(* Logix 5000 AddOnInstructionDefinition export Banner_QS18E_PD_v4; software revision 33.00 *)

TYPE Banner_QS18E_PDIO_v4 :   // Process Data for a QS18E sensors. This will include event information.
STRUCT
   Output_State : SINT;   // 0 = Inactive, 1 = Active
   Health_Signal : SINT;   // 0 = Marginal or Worse, 1 = Healthy
   Marginal_Light_State : SINT;   // 1 = Sensor is Marginal Light
   Marginal_Dark_State : SINT;   // 1 = Sensor is Marginal Dark
   Normalized_Signal_Strength : INT;
   Signal : DINT;   // Raw ADC Value
   Count : DINT;   // The output event count
   Duration : DINT;   // The output event duration
   Events_per_Minute : DINT;
   Emitter_LED : SINT;   // 0 = LED Emitter On, 1 = LED Emitter Off.
   Emitter_Status : SINT;   // 0 = Emitter enabled, 1 = Emitter disabled. Only active on QS18EK6E and QS18EK6EV models.
   PDI_DT : SINT[6];
   PDO_DT : SINT[2];
END_STRUCT
END_TYPE

ADD_ON_INSTRUCTION Banner_QS18E_PD_v4   (* revision 4.0, vendor Banner Engineering *)
// Take raw process data and convert it to usable values.
// Revision note:
// Added functionality for Emitter and Reciever QS18E models.
VAR_IN_OUT
   Process_Data : Banner_QS18E_PDIO_v4; {required}
END_VAR
VAR_INPUT
   PDI_Configuration : SINT; {required}
   Byte_Swap : BOOL; {required}
END_VAR
VAR
   Temp_iByte : SINT[4]; {access None}
END_VAR

ROUTINE Logic   (* ladder *)
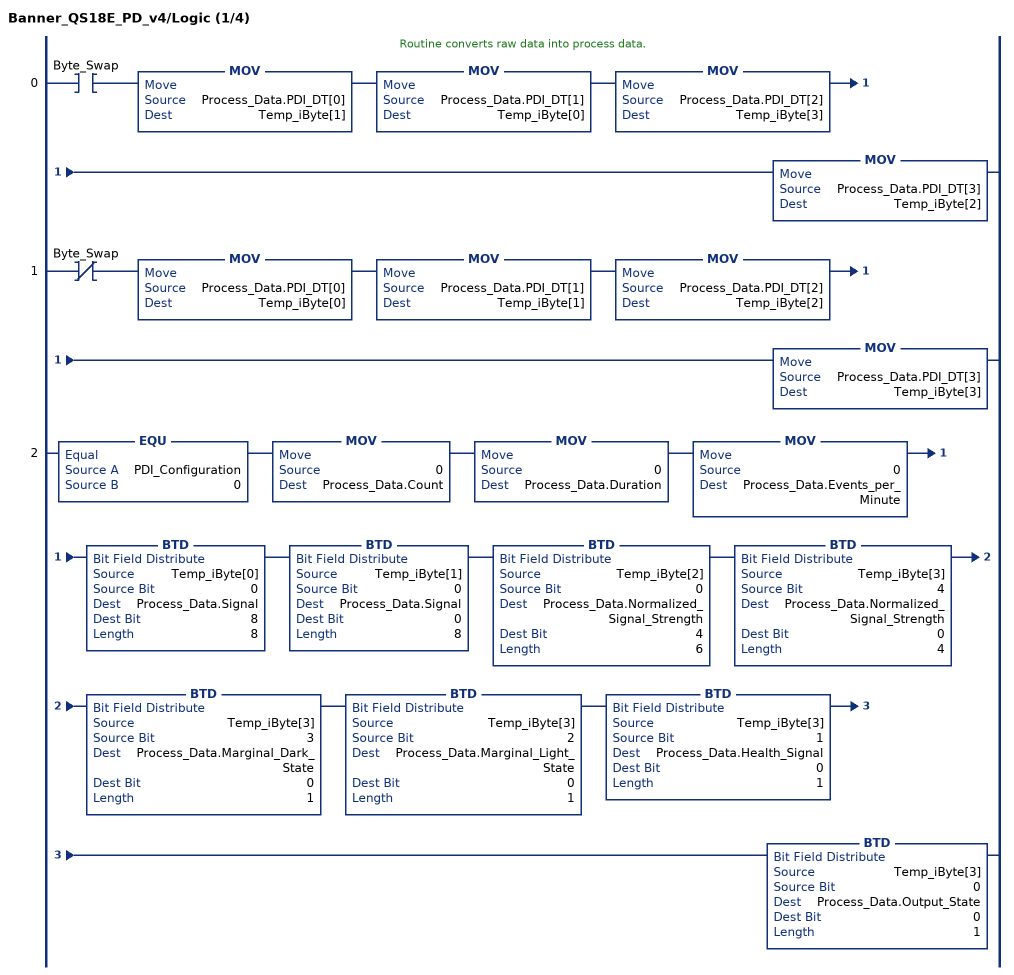
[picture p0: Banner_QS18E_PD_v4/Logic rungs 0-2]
   // Routine converts raw data into process data.
   0: XIC(Byte_Swap)MOV(Process_Data.PDI_DT[0],Temp_iByte[1])MOV(Process_Data.PDI_DT[1],Temp_iByte[0])MOV(Process_Data.PDI_DT[2],Temp_iByte[3])MOV(Process_Data.PDI_DT[3],Temp_iByte[2]);
   1: XIO(Byte_Swap)MOV(Process_Data.PDI_DT[0],Temp_iByte[0])MOV(Process_Data.PDI_DT[1],Temp_iByte[1])MOV(Process_Data.PDI_DT[2],Temp_iByte[2])MOV(Process_Data.PDI_DT[3],Temp_iByte[3]);
   2: EQU(PDI_Configuration,0)MOV(0,Process_Data.Count)MOV(0,Process_Data.Duration)MOV(0,Process_Data.Events_per_Minute)BTD(Temp_iByte[0],0,Process_Data.Signal,8,8)BTD(Temp_iByte[1],0,Process_Data.Signal,0,8)BTD(Temp_iByte[2],0,Process_Data.Normalized_Signal_Strength,4,6)BTD(Temp_iByte[3],4,Process_Data.Normalized_Signal_Strength,0,4)BTD(Temp_iByte[3],3,Process_Data.Marginal_Dark_State,0,1)BTD(Temp_iByte[3],2,Process_Data.Marginal_Light_State,0,1)BTD(Temp_iByte[3],1,Process_Data.Health_Signal,0,1)BTD(Temp_iByte[3],0,Process_Data.Output_State,0,1);
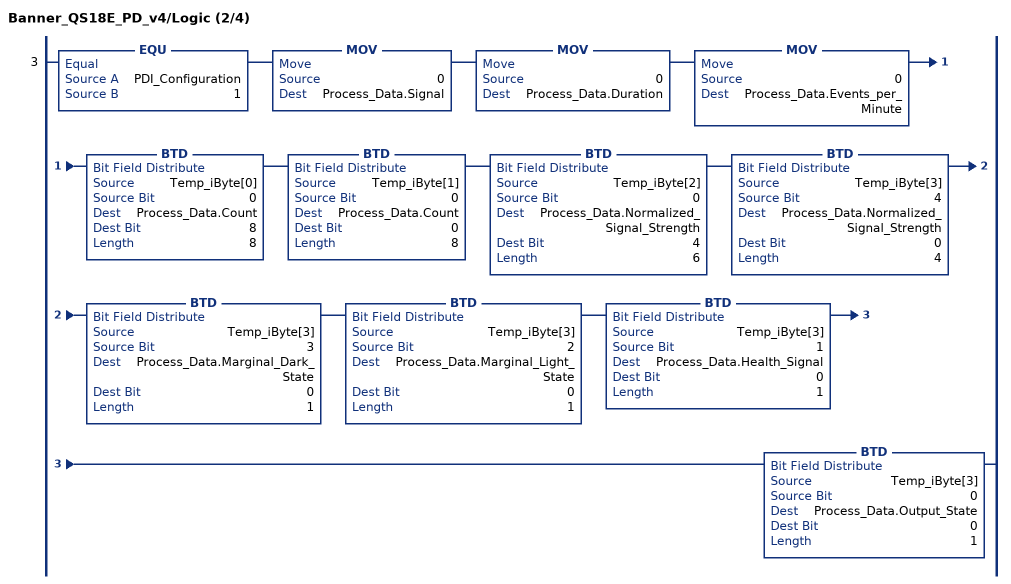
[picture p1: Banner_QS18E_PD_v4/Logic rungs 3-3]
   3: EQU(PDI_Configuration,1)MOV(0,Process_Data.Signal)MOV(0,Process_Data.Duration)MOV(0,Process_Data.Events_per_Minute)BTD(Temp_iByte[0],0,Process_Data.Count,8,8)BTD(Temp_iByte[1],0,Process_Data.Count,0,8)BTD(Temp_iByte[2],0,Process_Data.Normalized_Signal_Strength,4,6)BTD(Temp_iByte[3],4,Process_Data.Normalized_Signal_Strength,0,4)BTD(Temp_iByte[3],3,Process_Data.Marginal_Dark_State,0,1)BTD(Temp_iByte[3],2,Process_Data.Marginal_Light_State,0,1)BTD(Temp_iByte[3],1,Process_Data.Health_Signal,0,1)BTD(Temp_iByte[3],0,Process_Data.Output_State,0,1);
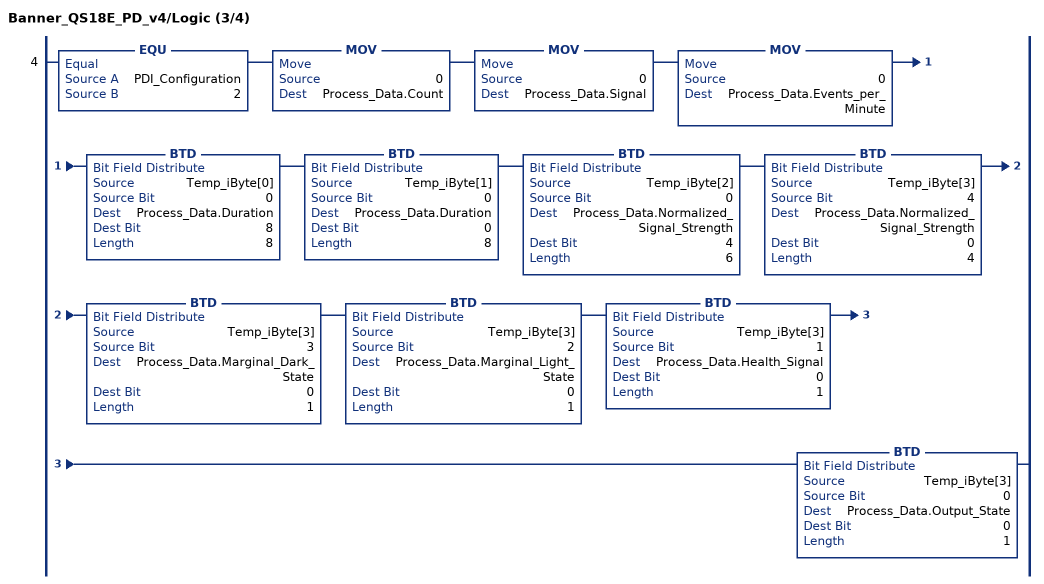
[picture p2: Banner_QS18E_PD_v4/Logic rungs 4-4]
   4: EQU(PDI_Configuration,2)MOV(0,Process_Data.Count)MOV(0,Process_Data.Signal)MOV(0,Process_Data.Events_per_Minute)BTD(Temp_iByte[0],0,Process_Data.Duration,8,8)BTD(Temp_iByte[1],0,Process_Data.Duration,0,8)BTD(Temp_iByte[2],0,Process_Data.Normalized_Signal_Strength,4,6)BTD(Temp_iByte[3],4,Process_Data.Normalized_Signal_Strength,0,4)BTD(Temp_iByte[3],3,Process_Data.Marginal_Dark_State,0,1)BTD(Temp_iByte[3],2,Process_Data.Marginal_Light_State,0,1)BTD(Temp_iByte[3],1,Process_Data.Health_Signal,0,1)BTD(Temp_iByte[3],0,Process_Data.Output_State,0,1);
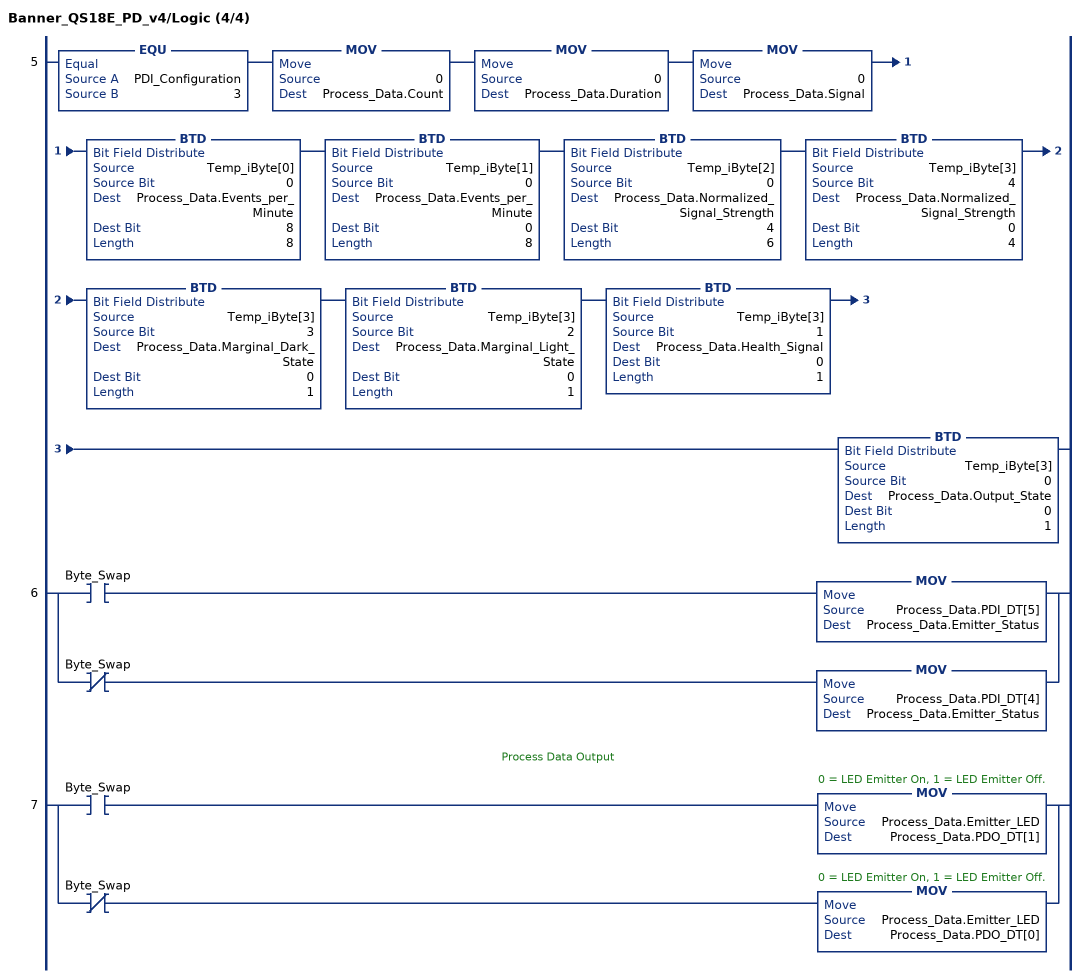
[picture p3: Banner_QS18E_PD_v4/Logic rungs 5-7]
   5: EQU(PDI_Configuration,3)MOV(0,Process_Data.Count)MOV(0,Process_Data.Duration)MOV(0,Process_Data.Signal)BTD(Temp_iByte[0],0,Process_Data.Events_per_Minute,8,8)BTD(Temp_iByte[1],0,Process_Data.Events_per_Minute,0,8)BTD(Temp_iByte[2],0,Process_Data.Normalized_Signal_Strength,4,6)BTD(Temp_iByte[3],4,Process_Data.Normalized_Signal_Strength,0,4)BTD(Temp_iByte[3],3,Process_Data.Marginal_Dark_State,0,1)BTD(Temp_iByte[3],2,Process_Data.Marginal_Light_State,0,1)BTD(Temp_iByte[3],1,Process_Data.Health_Signal,0,1)BTD(Temp_iByte[3],0,Process_Data.Output_State,0,1);
   6: [XIC(Byte_Swap) MOV(Process_Data.PDI_DT[5],Process_Data.Emitter_Status) ,XIO(Byte_Swap) MOV(Process_Data.PDI_DT[4],Process_Data.Emitter_Status) ];
   // Process Data Output
   7: [XIC(Byte_Swap) MOV(Process_Data.Emitter_LED,Process_Data.PDO_DT[1]) ,XIO(Byte_Swap) MOV(Process_Data.Emitter_LED,Process_Data.PDO_DT[0]) ];
END_ROUTINE
END_ADD_ON_INSTRUCTION
